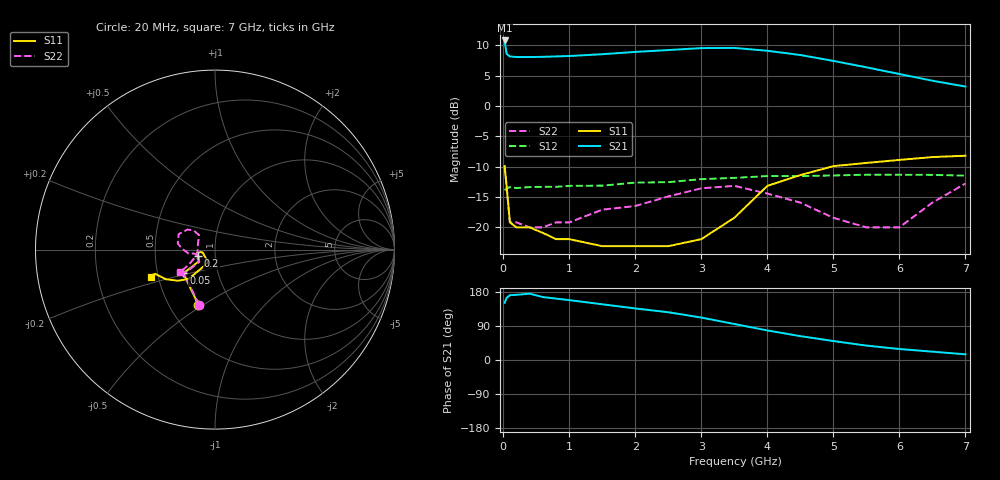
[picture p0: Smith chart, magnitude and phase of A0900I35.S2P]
!  MSA-0900 S PARAMETERS
!  Id=35mA  LAST UPDATED 07-27-92
# ghz s ma r 50
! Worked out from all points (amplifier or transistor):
!   20 points, 20 MHz to 7 GHz, reference 50 ohm
!   highest |S21| = 10.8 dB at 20 MHz (marker M1)
!   |S21| within 3 dB of that: start of sweep to 4.808 GHz
!   unconditionally stable (mu >= 1): 37.22 MHz to 2.991 GHz; 5.12 GHz to end of sweep
!   at 200 MHz: K = 1.19, MAG = 8.2 dB, |S12| = -13.5 dB
!   at 2.5 GHz: K = 1.04, MAG = 9.6 dB, |S12| = -12.5 dB
!   at 7 GHz: K = 1.17, MAG = 4.9 dB, |S12| = -11.5 dB
!   S11 on the Smith chart (normalised r, x): 20 MHz: 0.70, -0.47; 50 MHz: 0.68, -0.19; 200 MHz: 0.83, -0.06; 7 GHz: 0.45, -0.16
0.02  0.32 -107.0  3.48 151.0  0.203 17.0  0.32 -106.0
0.05  0.22 -143.0  2.7 164.0  0.209 6.0  0.22 -142.0
0.1  0.11 -144.0  2.57 171.0  0.215 3.0  0.11 -142.0
0.2  0.1 -160.0  2.54 172.0  0.211 1.0  0.11 -158.0
0.4  0.1 -171.0  2.54 175.0  0.215 2.0  0.1 -166.0
0.6  0.09 -170.0  2.55 166.0  0.216 1.0  0.1 -166.0
0.8  0.08 -170.0  2.57 162.0  0.216 1.0  0.11 -166.0
1  0.08 -170.0  2.59 158.0  0.22 1.0  0.11 -167.0
1.5  0.07 -166.0  2.68 147.0  0.221 1.0  0.14 -172.0
2  0.07 -138.0  2.8 136.0  0.234 1.0  0.15 -172.0
2.5  0.07 -131.0  2.9 126.0  0.236 1.0  0.18 179.0
3  0.08 -119.0  3.01 112.0  0.25 1.0  0.21 171.0
3.5  0.12 -125.0  3.02 95.0  0.256 -1.0  0.22 157.0
4  0.22 -132.0  2.86 78.0  0.265 -3.0  0.19 144.0
4.5  0.27 -140.0  2.64 63.0  0.265 -5.0  0.16 138.0
5  0.32 -149.0  2.36 50.0  0.268 -6.0  0.12 138.0
5.5  0.34 -154.0  2.09 38.0  0.272 -6.0  0.1 162.0
6  0.36 -158.0  1.84 29.0  0.272 -6.0  0.1 -166.0
6.5  0.38 -158.0  1.62 22.0  0.271 -6.0  0.16 -151.0
7  0.39 -157.0  1.45 15.0  0.267 -6.0  0.23 -147.0
